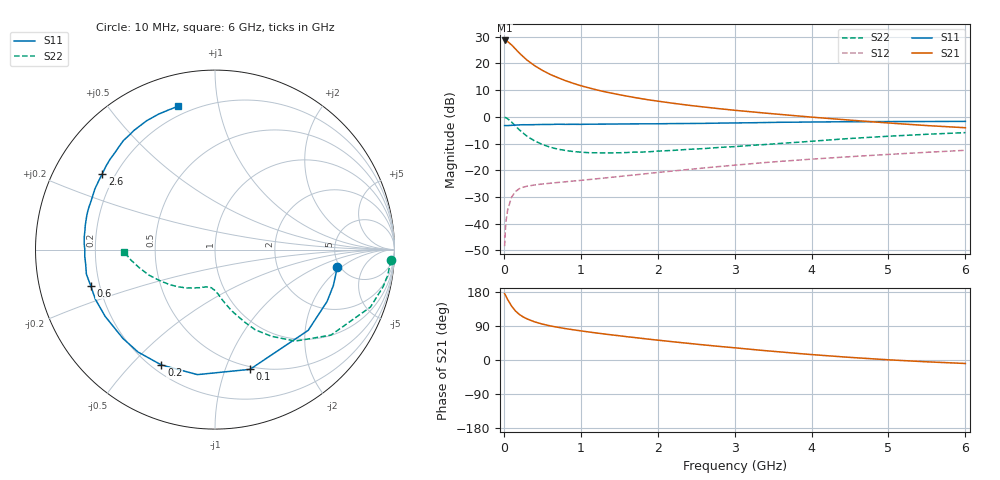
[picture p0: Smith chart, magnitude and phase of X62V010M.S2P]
! SIEMENS Small Signal Semiconductors
! BFP193W
! Si NPN RF Bipolar Junction Transistor in SOT343
! VCE = 2 V  IC = 10 mA
! Common Emitter S-Parameters:  April 1994
# GHz  S  MA  R  50
!  f  S11  S21  S12  S22
! GHz  MAG  ANG  MAG  ANG  MAG  ANG  MAG  ANG
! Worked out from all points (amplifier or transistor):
!   40 points, 10 MHz to 6 GHz, reference 50 ohm
!   highest |S21| = 28.6 dB at 10 MHz (marker M1)
!   |S21| within 3 dB of that: start of sweep to 145 MHz
!   unconditionally stable (mu >= 1): 1.265 GHz to 4.274 GHz
!   at 200 MHz: K = 0.22, MSG = 25.4 dB, |S12| = -26.9 dB
!   at 1.5 GHz: K = 1.07, MAG = 13.7 dB, |S12| = -22.3 dB
!   at 6 GHz: K = 0.93, MSG = 4.2 dB, |S12| = -12.5 dB
!   lowest NFmin = 1.30 dB at 450 MHz
!   S11 on the Smith chart (normalised r, x): 10 MHz: 4.72, -1.78; 100 MHz: 0.47, -1.22; 200 MHz: 0.24, -0.61; 600 MHz: 0.16, -0.14; 2.6 GHz: 0.15, +0.30; 6 GHz: 0.15, +0.77
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0.01  0.6884 -8.3  27 174.9  0.0038 87.2  0.9824 -3.4
0.02  0.6892 -16.9  26.95 171.6  0.0077 81.6  0.9728 -8.5
0.03  0.688 -24.9  26.69 167.5  0.0116 79.1  0.959 -12.5
0.05  0.6871 -40.9  25.7 159.4  0.0183 71.6  0.9232 -20.3
0.1  0.6951 -73.7  22.3 142.6  0.0313 57.6  0.8026 -36.4
0.15  0.7034 -98.0  18.79 129.6  0.0399 47.4  0.6787 -48.7
0.2  0.7088 -114.9  15.77 120.5  0.0452 41.2  0.5755 -57.0
0.25  0.7139 -126.9  13.5 113.8  0.0483 37.0  0.4993 -63.4
0.3  0.7128 -136.0  11.61 108.6  0.0504 34.4  0.4358 -67.8
0.4  0.7162 -148.7  9.099 100.7  0.0532 31.5  0.3552 -74.6
0.5  0.7216 -157.4  7.446 94.8  0.0555 30.7  0.3052 -79.3
0.6  0.7214 -163.9  6.274 90.2  0.0572 30.8  0.2717 -83.1
0.8  0.7252 -173.3  4.772 82.9  0.061 32.5  0.2352 -88.5
1.1  0.73 177.2  3.517 74.1  0.067 35.7  0.2139 -95.1
1.3  0.7323 171.6  2.983 68.8  0.0715 37.9  0.2122 -99.1
1.6  0.7393 164.9  2.45 61.4  0.0794 41.0  0.2152 -104.5
2.2  0.7497 153.2  1.801 48.1  0.0972 44.7  0.236 -115.8
2.6  0.7567 146.1  1.532 39.8  0.1105 45.7  0.2552 -123.4
3.2  0.7761 136.0  1.252 28.4  0.1322 45.4  0.2916 -134.6
4.5  0.8126 118.0  0.87 6.9  0.18 40.6  0.3947 -158.9
5.5  0.8197 108.7  0.688 -4.8  0.2174 35.6  0.4731 -173.1
6  0.8249 104.3  0.627 -9.2  0.237 33.0  0.5081 -178.8
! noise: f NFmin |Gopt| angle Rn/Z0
0.45  1.3  0.22  143  0.11
0.9  1.3  0.34  160  0.11
1.8  2.05  0.54  -153  0.14
